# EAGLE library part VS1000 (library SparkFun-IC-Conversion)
VS1000D Ogg Vorbis Player IC with USB and NAND FLASH Interface 12 MHz LQFP-48 Datasheet SparkFun Products Storefront component: Ogg Vorbis Codec IC - VS1000D (COM-08300)
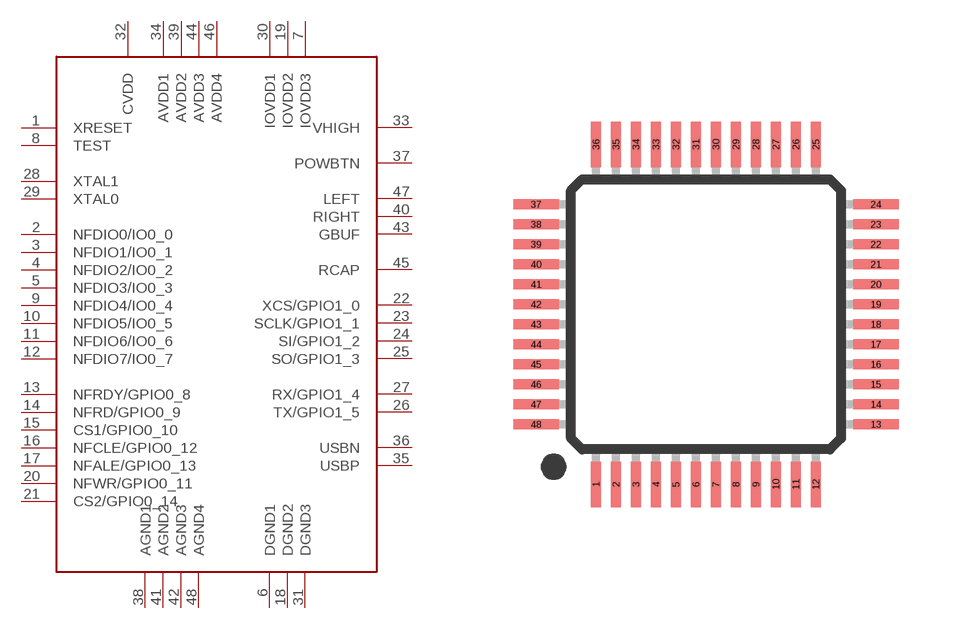
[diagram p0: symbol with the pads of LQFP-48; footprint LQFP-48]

Designator prefix -

## VS1000 (PROD_ID: LPA-12743; VALUE: VS1000D)  [LQFP-48]
1  XRESET
2  NFDIO0/IO0_0
3  NFDIO1/IO0_1
4  NFDIO2/IO0_2
5  NFDIO3/IO0_3
6  DGND1
7  IOVDD3
8  TEST
9  NFDIO4/IO0_4
10  NFDIO5/IO0_5
11  NFDIO6/IO0_6
12  NFDIO7/IO0_7
13  NFRDY/GPIO0_8
14  NFRD/GPIO0_9
15  CS1/GPIO0_10
16  NFCLE/GPIO0_12
17  NFALE/GPIO0_13
18  DGND2
19  IOVDD2
20  NFWR/GPIO0_11
21  CS2/GPIO0_14
22  XCS/GPIO1_0
23  SCLK/GPIO1_1
24  SI/GPIO1_2
25  SO/GPIO1_3
26  TX/GPIO1_5
27  RX/GPIO1_4
28  XTAL1
29  XTAL0
30  IOVDD1
31  DGND3
32  CVDD
33  VHIGH
34  AVDD1
35  USBP
36  USBN
37  POWBTN
38  AGND1
39  AVDD2
40  RIGHT
41  AGND2
42  AGND3
43  GBUF
44  AVDD3
45  RCAP
46  AVDD4
47  LEFT
48  AGND4

## Footprint LQFP-48 (pad centres in mm)
LQFP -48 Specifications: Pin count: 48 Example device(s): VS1000
smd 0.254 x 1.143: 1 -2.75,-4.25; 2 -2.25,-4.25; 3 -1.75,-4.25; 4 -1.25,-4.25; 5 -0.75,-4.25; 6 -0.25,-4.25; 7 0.25,-4.25; 8 0.75,-4.25; 9 1.25,-4.25; 10 1.75,-4.25; 11 2.25,-4.25; 12 2.75,-4.25; 25 2.75,4.25; 26 2.25,4.25; 27 1.75,4.25; 28 1.25,4.25; 29 0.75,4.25; 30 0.25,4.25; 31 -0.25,4.25; 32 -0.75,4.25; 33 -1.25,4.25; 34 -1.75,4.25; 35 -2.25,4.25; 36 -2.75,4.25
smd 1.143 x 0.254: 13 4.25,-2.75; 14 4.25,-2.25; 15 4.25,-1.75; 16 4.25,-1.25; 17 4.25,-0.75; 18 4.25,-0.25; 19 4.25,0.25; 20 4.25,0.75; 21 4.25,1.25; 22 4.25,1.75; 23 4.25,2.25; 24 4.25,2.75; 37 -4.25,2.75; 38 -4.25,2.25; 39 -4.25,1.75; 40 -4.25,1.25; 41 -4.25,0.75; 42 -4.25,0.25; 43 -4.25,-0.25; 44 -4.25,-0.75; 45 -4.25,-1.25; 46 -4.25,-1.75; 47 -4.25,-2.25; 48 -4.25,-2.75

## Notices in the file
Licensing: Creative Commons ShareAlike 4.0 International - https://creativecommons.org/licenses/by-sa/4.0
